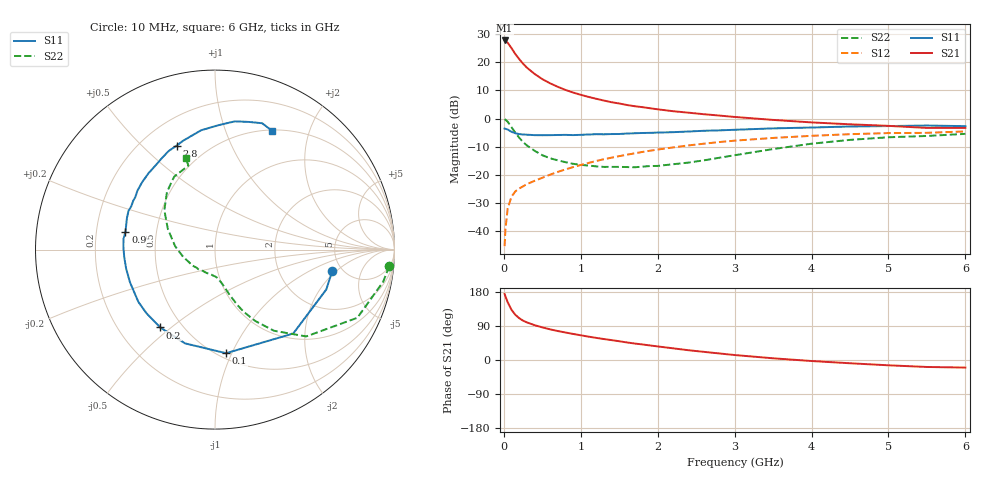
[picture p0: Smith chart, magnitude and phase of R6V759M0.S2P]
! SIEMENS Small Signal Semiconductors
! BFR193
! Si NPN RF Bipolar Junction Transistor in SOT23
! VCE = 0.75 V  IC = 9 mA
! Common Emitter S-Parameters:  May  1996
# GHz  S  MA  R  50
!  f  S11  S21  S12  S22
! GHz  MAG  ANG  MAG  ANG  MAG  ANG  MAG  ANG
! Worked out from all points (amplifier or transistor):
!   36 points, 10 MHz to 6 GHz, reference 50 ohm
!   highest |S21| = 27.8 dB at 10 MHz (marker M1)
!   |S21| within 3 dB of that: start of sweep to 106.4 MHz
!   unconditionally stable (mu >= 1): 717.9 MHz to 2.293 GHz
!   at 250 MHz: K = 0.62, MSG = 21.8 dB, |S12| = -24.1 dB
!   at 1.4 GHz: K = 1.06, MAG = 8.4 dB, |S12| = -13.9 dB
!   at 6 GHz: K = 0.98, MSG = 0.6 dB, |S12| = -4.6 dB
!   S11 on the Smith chart (normalised r, x): 10 MHz: 4.18, -1.76; 100 MHz: 0.55, -0.95; 200 MHz: 0.38, -0.46; 900 MHz: 0.33, +0.09; 2.8 GHz: 0.34, +0.64; 6 GHz: 0.51, +1.47
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0.01  0.6643 -10.2  24.45 174.2  0.0054 83.9  0.9749 -5.5
0.02  0.6587 -19.7  23.89 168.3  0.0105 83.5  0.9541 -10.8
0.05  0.6393 -47.0  22.25 152.4  0.0253 70.0  0.8794 -25.6
0.1  0.5805 -83.9  17.86 132.4  0.0411 57.6  0.7015 -43.6
0.15  0.5485 -107.7  13.99 119.2  0.0508 51.8  0.5589 -54.0
0.2  0.5303 -125.1  11.39 110.3  0.0572 50.3  0.4565 -60.6
0.25  0.5211 -137.2  9.441 103.8  0.0625 49.7  0.3819 -65.2
0.3  0.5169 -145.7  8.031 99.2  0.0684 50.3  0.333 -68.0
0.4  0.5076 -158.9  6.208 91.9  0.0784 52.2  0.2675 -71.9
0.5  0.5064 -168.0  5.023 86.1  0.0887 54.1  0.2232 -75.2
0.6  0.5074 -175.3  4.242 81.0  0.1006 55.8  0.1973 -77.8
0.7  0.5108 178.3  3.675 76.5  0.1126 56.8  0.1811 -80.3
0.9  0.5086 168.8  2.903 68.8  0.1373 57.5  0.1572 -85.7
1.1  0.5211 160.3  2.427 61.7  0.1627 57.6  0.1463 -93.2
1.3  0.5253 152.6  2.092 55.3  0.1896 56.6  0.1383 -101.0
1.6  0.5427 142.8  1.743 46.3  0.228 54.3  0.1375 -114.8
2.2  0.5731 125.7  1.352 30.8  0.3072 47.4  0.1543 -145.1
2.8  0.6172 110.3  1.132 17.3  0.3824 38.8  0.2011 -177.3
3.5  0.6695 96.6  0.947 4.5  0.4529 27.8  0.2871 156.3
4.5  0.723 81.2  0.791 -8.6  0.5281 13.1  0.4182 129.8
5.5  0.7515 69.5  0.682 -18.4  0.5582 -1.1  0.491 107.6
6  0.7339 64.3  0.683 -20.0  0.5909 -5.3  0.5353 107.6
